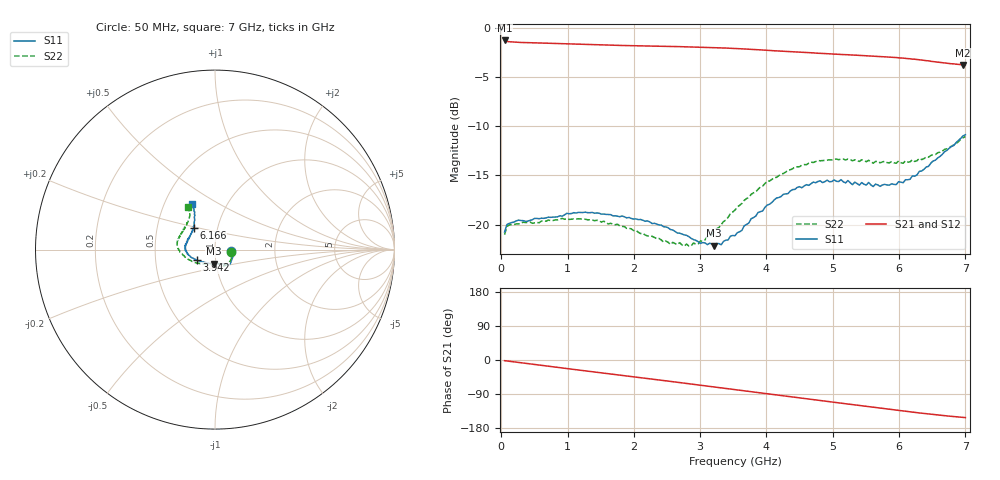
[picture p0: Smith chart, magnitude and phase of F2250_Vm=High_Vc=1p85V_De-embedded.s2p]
! Integrated Device Technology
! Corporate Headquarters
! 6024 Silver Creek Valley Road
! San Jose, CA 95138  USA
! Phone:  1-408-284-8200
! Toll Free:  1-800-223-1366
! Webpage:  http://www.idt.com/
! Timing and RF Division
! 515 Groton Road, Suite 102
! Westford, MA 01886-6024
! Device:  F2250
! Description: Voltage Variable RF Attenuator
! Frequency:  50.0 -  6000.00 MHz
! Package:  3x3 mm Thin QFN Plastic Package: 16 pin
! Ports:  2 RF, 3 DC
!  Pin  1  = GND
!  Pin  2  = NC
!  Pin  3  = RF1  = Port 1
!  Pin  4  = NC
!  Pin  5  = GND
!  Pin  6  = GND
!  Pin  7  = GND
!  Pin  8  = GND
!  Pin  9  = NC
!  Pin 10  = RF2  = Port 2
!  Pin 11  = NC
!  Pin 12  = GND
!  Pin 13  = GND
!  Pin 14  = VCNTRL
!  Pin 15  = VDD
!  Pin 16  = VMODE
! Vcntrl:  1.850 Volts
! Vmode:  +3.300 Volts
! Vdd:  +3.30  Volts
! Current:  1.324 mA
! Data:  The device was measured on a the F2250 evaluation board which has
!  individual transmission lines to the RF pins.  Data was collected
!  using a calibrated network analyzer.  The evaluation board was
!  de-embedded using a TRL calibration technique.
!  The reference plane is the edge of the package pin.
! Misc:  SN 10
!  Action Tracker AT0258
! Date Measured:  2014-11-26
! Date:  2015-10-15  MJV
! Note:
!  Integrated Device Technology supplies this data as a sample of measured
!  data at the package pin for this product.  Your particular data for this
!  product may vary.
!  Data was taken at 25 degrees C.
!  Integrated Device Technology reserves the right to change this data at anytime.
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# GHz S dB R 50
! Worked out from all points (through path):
!   201 points, 50 MHz to 7 GHz, reference 50 ohm
!   highest |S21| = -1.29 dB at 50 MHz (marker M1); lowest = -3.8 dB at 6.965 GHz (marker M2)
!   group delay of S21, straight-line fit = 61.1 ps
!   lowest |S11| = -22.1 dB at 3.212 GHz (marker M3), VSWR 1.17, Z = 48.7 - j7.63 ohm
!   |S11| at or under -10 dB: start of sweep to end of sweep
!   |S22| runs from -22.2 to -11.1 dB; largest |S21 - S12| = 0.0018
!   S11 on the Smith chart (normalised r, x): 50 MHz: 1.20, -0.02; 3.942 GHz: 0.81, -0.09; 6.166 GHz: 0.77, +0.19; 7 GHz: 0.69, +0.38
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0.05  -20.75 -6.0  -1.29 -1.8  -1.29 -1.8  -21.02 -7.2
0.08475  -20.00 -5.8  -1.38 -2.5  -1.38 -2.5  -20.19 -6.7
0.1195  -19.88 -6.5  -1.42 -3.3  -1.42 -3.3  -20.03 -6.7
0.6755  -19.32 -27.0  -1.57 -15.7  -1.57 -15.7  -19.66 -30.7
1.2315  -18.77 -43.8  -1.69 -27.9  -1.69 -27.9  -19.45 -52.6
1.75275  -19.14 -50.8  -1.79 -39.1  -1.78 -39.1  -19.96 -62.7
2.37825  -20.04 -53.4  -1.88 -52.6  -1.88 -52.6  -21.41 -71.8
2.552  -20.50 -57.0  -1.89 -56.5  -1.89 -56.5  -22.01 -78.3
2.86475  -21.40 -67.8  -1.94 -63.5  -1.94 -63.5  -22.16 -95.0
3.21225  -22.13 -95.4  -2.01 -71.3  -2.01 -71.3  -20.65 -121.3
3.525  -21.13 -123.8  -2.11 -78.4  -2.11 -78.5  -18.53 -140.0
3.942  -18.61 -150.9  -2.26 -87.8  -2.26 -87.8  -16.09 -159.3
4.1505  -17.30 -159.9  -2.35 -92.4  -2.35 -92.5  -15.20 -167.6
4.4285  -16.42 -169.2  -2.45 -98.6  -2.46 -98.6  -14.14 -176.1
4.7065  -15.68 -177.6  -2.55 -104.7  -2.55 -104.7  -13.69 177.5
5.22775  -15.52 168.4  -2.74 -116.2  -2.74 -116.2  -13.34 165.8
5.29725  -15.95 166.0  -2.76 -117.6  -2.76 -117.7  -13.52 164.5
5.85325  -15.98 146.7  -2.98 -129.8  -2.98 -129.9  -13.72 150.0
6.166  -15.39 134.2  -3.15 -136.7  -3.15 -136.8  -13.63 141.4
6.54825  -13.45 122.9  -3.45 -144.5  -3.45 -144.6  -12.88 129.0
6.96525  -10.98 117.0  -3.78 -151.5  -3.79 -151.6  -11.18 123.2
7  -10.87 116.6  -3.78 -151.9  -3.79 -152.0  -11.06 122.3
